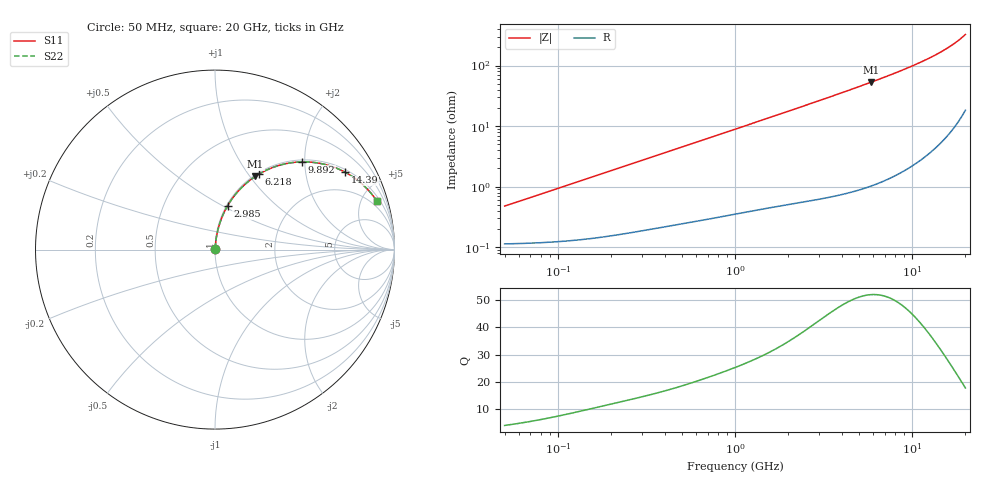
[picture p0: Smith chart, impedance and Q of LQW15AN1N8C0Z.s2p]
!Murata Part Number: LQW15AN1N8C0Z
!These Parameters are Measured in Series Mode Connection
!  o--[Z]--o
!Port1  Port2
!  o-------o
!Freq. Start=50[MHz] Stop=20[GHz], 401[Steps]
# Hz S RI R 50
!Freq.(Hz) S11(Real) S11(Imag) S21(Real) S21(Imag) S12(Real) S12(Imag) S22(Real) S22(Imag)
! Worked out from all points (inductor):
!   401 points, 50 MHz to 20 GHz, reference 50 ohm
!   read as one part in series: L = 1.48 nH near 51.52 MHz
!   highest Q = 51.9 at 5.856 GHz (marker M1), where L = 1.44 nH
!   S11 on the Smith chart (normalised r, x): 50 MHz: 1.00, +0.01; 2.985 GHz: 1.01, +0.53; 6.218 GHz: 1.02, +1.13; 9.892 GHz: 1.04, +1.94; 14.39 GHz: 1.10, +3.29; 20 GHz: 1.37, +6.52
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5e7  0.00115 0.00465  0.9988 -0.00465  0.9988 -0.00465  0.00115 0.00465
6.166548e7  0.00118 0.00573  0.9988 -0.00573  0.9988 -0.00573  0.00118 0.00573
1.364002e8  0.00149 0.0126  0.9985 -0.0126  0.9985 -0.0126  0.00149 0.0126
3.721004e8  0.00321 0.0336  0.9968 -0.0336  0.9968 -0.0336  0.00321 0.0336
6.380365e8  0.00598 0.0566  0.994 -0.0566  0.994 -0.0566  0.00598 0.0566
1e9  0.0112 0.0875  0.9888 -0.0875  0.9888 -0.0875  0.0112 0.0875
1.689197e9  0.026 0.1443  0.974 -0.1443  0.974 -0.1443  0.026 0.1443
2.728004e9  0.0595 0.2246  0.9405 -0.2246  0.9405 -0.2246  0.0595 0.2246
2.98453e9  0.0698 0.2432  0.9302 -0.2432  0.9302 -0.2432  0.0698 0.2432
3.626126e9  0.0984 0.2872  0.9016 -0.2872  0.9016 -0.2872  0.0984 0.2872
4.275624e9  0.1313 0.3277  0.8687 -0.3277  0.8687 -0.3277  0.1313 0.3277
5.041459e9  0.1744 0.3698  0.8256 -0.3698  0.8256 -0.3698  0.1744 0.3698
5.856089e9  0.2239 0.4073  0.7761 -0.4073  0.7761 -0.4073  0.2239 0.4073
6.217679e9  0.2468 0.4216  0.7532 -0.4216  0.7532 -0.4216  0.2468 0.4216
7.442007e9  0.3266 0.4592  0.6734 -0.4592  0.6734 -0.4592  0.3266 0.4592
8.644534e9  0.4056 0.4808  0.5944 -0.4808  0.5944 -0.4808  0.4056 0.4808
9.892087e9  0.4852 0.4888  0.5148 -0.4888  0.5148 -0.4888  0.4852 0.4888
1.201863e10  0.6092 0.4753  0.3908 -0.4753  0.3908 -0.4753  0.6092 0.4753
1.438523e10  0.7247 0.4314  0.2753 -0.4314  0.2753 -0.4314  0.7247 0.4314
1.696185e10  0.8218 0.3633  0.1782 -0.3633  0.1782 -0.3633  0.8218 0.3633
1.88369e10  0.8751 0.3072  0.1249 -0.3072  0.1249 -0.3072  0.8751 0.3072
2e10  0.9016 0.2711  0.0984 -0.2711  0.0984 -0.2711  0.9016 0.2711
